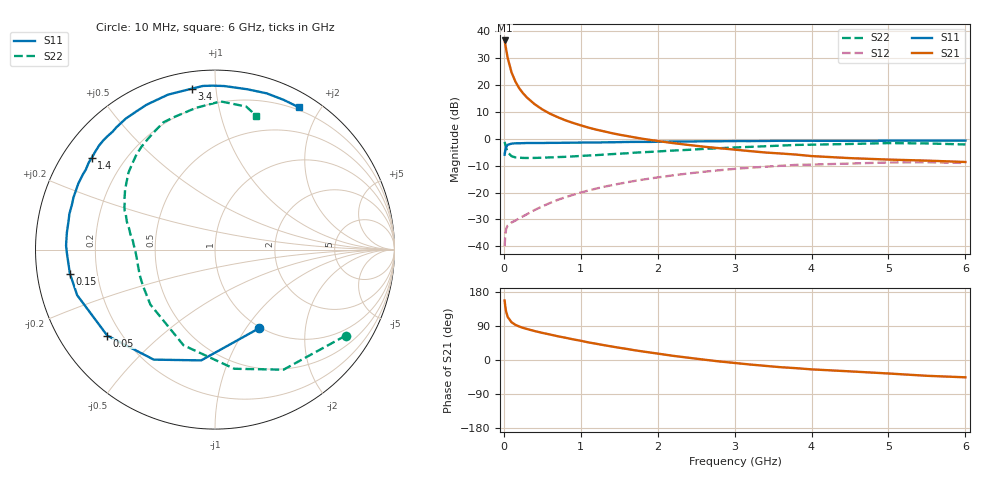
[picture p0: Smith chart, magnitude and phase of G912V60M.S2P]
! SIEMENS Small Signal Semiconductors
! BFG235
! Si NPN RF Bipolar Junction Transistor in SOT223
! VCE = 12 V  IC = 60 mA
! Common Emitter S-Parameters:  July  1994
# GHz  S  MA  R  50
!  f  S11  S21  S12  S22
! GHz  MAG  ANG  MAG  ANG  MAG  ANG  MAG  ANG
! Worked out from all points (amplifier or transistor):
!   40 points, 10 MHz to 6 GHz, reference 50 ohm
!   highest |S21| = 36.5 dB at 10 MHz (marker M1)
!   |S21| within 3 dB of that: start of sweep to 28.1 MHz
!   unconditionally stable (mu >= 1): 515.5 MHz to 1.401 GHz
!   at 200 MHz: K = 0.68, MSG = 24.1 dB, |S12| = -29.5 dB
!   at 1.5 GHz: K = 0.98, MSG = 9.1 dB, |S12| = -16.7 dB
!   at 6 GHz: K = 0.91, MSG = 0.2 dB, |S12| = -9.0 dB
!   S11 on the Smith chart (normalised r, x): 10 MHz: 0.98, -1.15; 50 MHz: 0.15, -0.34; 150 MHz: 0.10, -0.08; 1.4 GHz: 0.09, +0.33; 3.4 GHz: 0.09, +0.86; 6 GHz: 0.17, +1.74
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0.01  0.5024 -60.9  66.49 156.9  0.0101 67.1  0.8712 -33.4
0.02  0.622 -97.1  55.19 139.6  0.0171 53.3  0.7702 -60.3
0.03  0.7016 -119.1  45.34 127.5  0.0211 44.3  0.6726 -80.8
0.05  0.7681 -141.4  31.44 113.6  0.0244 33.9  0.5612 -108.2
0.1  0.8089 -161.7  17.01 99.6  0.0278 31.8  0.4725 -139.7
0.15  0.8192 -170.5  11.49 92.8  0.0301 35.2  0.4491 -153.5
0.2  0.8208 -174.9  8.624 88.4  0.0334 38.7  0.443 -161.1
0.25  0.8257 -178.8  6.943 84.8  0.0362 42.9  0.4391 -165.9
0.3  0.8301 178.4  5.806 81.9  0.0396 46.1  0.4382 -169.8
0.4  0.8307 173.5  4.368 76.4  0.0473 50.8  0.439 -174.6
0.5  0.831 169.4  3.488 71.6  0.0553 53.5  0.4429 -178.2
0.6  0.8352 166.3  2.909 67.3  0.0639 55.1  0.4489 178.7
0.7  0.8357 162.4  2.506 62.7  0.0731 56.3  0.4548 176.2
0.9  0.8422 156.7  1.957 54.5  0.0906 56.1  0.4682 172.0
1.1  0.8468 150.5  1.602 46.4  0.109 54.9  0.4863 167.8
1.4  0.8561 143.3  1.269 35.7  0.1364 51.7  0.5161 162.2
2.2  0.883 124.3  0.828 11.0  0.2084 39.0  0.6015 146.4
3.2  0.9016 102.6  0.587 -11.9  0.2886 19.4  0.7042 125.6
3.4  0.9057 98.3  0.553 -15.5  0.3012 15.1  0.7229 120.8
4.5  0.9112 78.6  0.435 -30.0  0.345 -6.8  0.7969 97.6
5.5  0.9178 65.3  0.391 -41.7  0.3645 -25.7  0.8156 77.7
6  0.9199 59.5  0.369 -45.7  0.3535 -32.4  0.78 72.8
